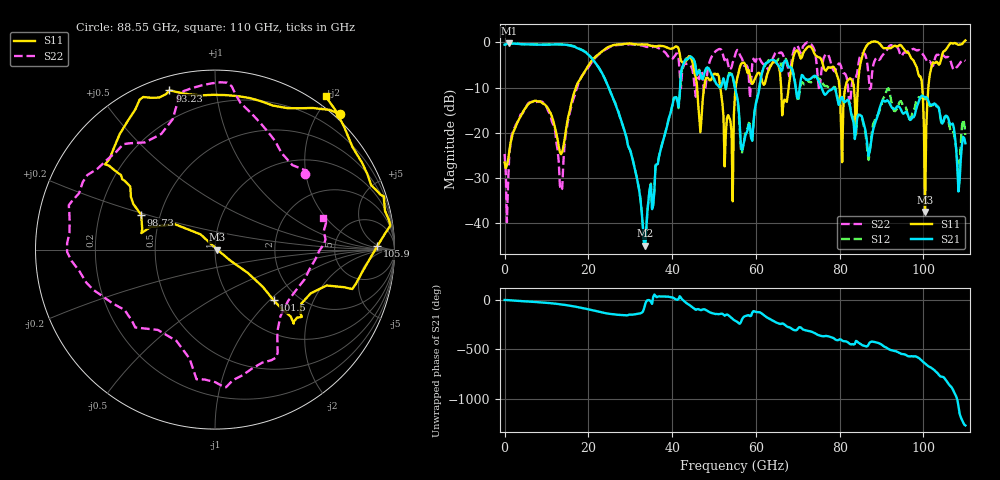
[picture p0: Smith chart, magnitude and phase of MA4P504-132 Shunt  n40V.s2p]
!Keysight Technologies,N5247B,US61255204,A.15.70.20
!Date: Friday, October 21, 2022 14:54:19
!Correction: S11(C  4-Port  )
!S31(C  4-Port  )
!S13(C  4-Port  )
!S33(C  4-Port  )
!S2P File: Measurements: S11, S31, S13, S33:
# Hz S  dB  R 50
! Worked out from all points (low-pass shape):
!   401 points, 10 MHz to 110 GHz, reference 50 ohm
!   highest |S21| = -0.19 dB at 1.11 GHz (marker M1); lowest = -45.1 dB at 33.56 GHz (marker M2)
!   |S21| within 3 dB of the highest: start of sweep to 20.5 GHz; 44.23 GHz to 44.59 GHz (358.8 MHz wide, 0.808 % of centre)
!   lowest |S11| = -37.6 dB at 100.4 GHz (marker M3), VSWR 1.03, Z = 51.3 - j0.0617 ohm
!   |S11| at or under -10 dB: start of sweep to 17.04 GHz; 45.97 GHz to 47.62 GHz (1.653 GHz wide, 3.53 % of centre); 51.49 GHz to 55.18 GHz (3.69 GHz wide, 6.92 % of centre)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
!   |S22| runs from -39.8 to 0.0 dB; largest |S21 - S12| = 0.25
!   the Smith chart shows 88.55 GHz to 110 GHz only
!   S11 on the Smith chart (normalised r, x): 88.55 GHz: -0.08, +2.28; 93.23 GHz: 0.06, +0.75; 98.73 GHz: 0.39, +0.19; 101.5 GHz: 1.53, -1.06; 105.9 GHz: 19, +4; 110 GHz: -0.12, +1.95
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1e7  -26.58 2.2  -0.49 -0.2  -0.48 -0.0  -24.71 -3.0
1.1099e9  -24.23 68.2  -0.19 -2.7  -0.17 -2.5  -25.08 102.4
8.534225e9  -13.09 74.2  -0.50 -23.6  -0.46 -23.4  -13.10 58.2
1.348378e10  -24.75 135.5  -0.45 -44.1  -0.38 -43.8  -32.80 -44.8
1.843332e10  -7.53 177.2  -1.67 -79.5  -1.61 -79.5  -7.44 -158.2
3.355695e10  -0.45 119.2  -45.06 -44.6  -45.16 -44.3  -0.87 122.8
3.685665e10  -0.74 117.4  -25.37 36.5  -25.21 36.3  -1.30 126.3
4.428098e10  -3.09 23.9  -3.14 -55.0  -3.31 -55.6  -5.10 74.8
4.84056e10  -7.79 -167.1  -5.55 -109.7  -5.56 -109.8  -6.63 135.2
5.5005e10  -11.48 -108.3  -9.97 151.3  -10.22 149.4  -2.94 168.0
5.692982e10  -4.49 -112.7  -22.96 -178.0  -23.22 -164.9  -4.33 156.9
6.6004e10  -9.69 -36.9  -6.36 118.4  -5.03 122.9  -2.18 48.1
7.342832e10  -1.36 138.1  -7.73 37.3  -8.44 35.6  -0.68 108.5
7.975275e10  -8.36 -164.8  -13.84 -43.1  -13.33 -44.3  -4.69 -142.8
8.855195e10  0.21 47.3  -17.53 -66.6  -16.65 -49.0  -3.64 40.0
9.185165e10  -1.28 90.5  -13.38 -139.3  -10.74 -133.7  -0.77 84.2
9.322652e10  -0.70 106.0  -14.74 -156.3  -15.25 -154.3  -0.83 98.0
9.872602e10  -6.84 154.8  -13.43 137.5  -12.21 137.1  -1.67 177.6
1.003759e11  -37.59 -2.6  -12.11 79.1  -12.60 80.7  -3.42 -157.0
1.014758e11  -7.29 -40.8  -13.78 43.0  -14.09 48.9  -4.14 -135.7
1.058754e11  -0.88 1.2  -16.71 -122.6  -17.20 -125.6  -3.21 -60.6
1.1e11  0.45 54.2  -22.34 172.4  -20.50 174.4  -4.08 16.2
